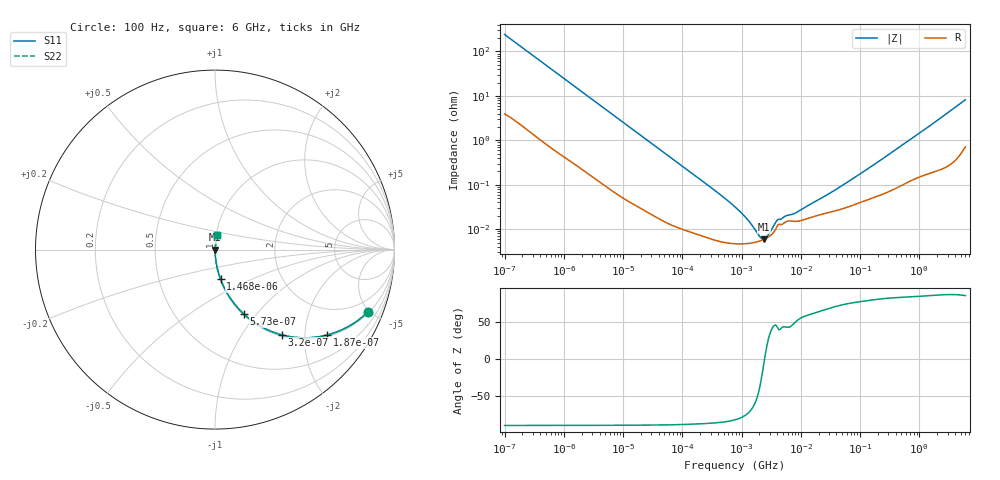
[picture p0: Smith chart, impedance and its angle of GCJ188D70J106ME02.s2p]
!Murata Part Number: GCJ188D70J106ME02
!These Parameters are Measured in Series Mode Connection
!Data Generated on Mar 13, 2026
!  o--ll--o
!Port1  Port2
!  o------o
!Operation Temp=25[degC], DC Bias Voltage=0[V]
!Freq. Start=100[Hz] Stop=6[GHz] 401[Steps]
# Hz S RI R 50
!Freq.(Hz) S11(Real) S11(Imag) S21(Real) S21(Imag) S12(Real) S12(Imag) S22(Real) S22(Imag)
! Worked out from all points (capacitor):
!   401 points, 100 Hz to 6 GHz, reference 50 ohm
!   read as one part in series: C = 6.56 uF near 109 Hz
!   lowest |Z| = 5.89 mohm at 2.373 MHz (marker M1)
!   series resonance near 2.443 MHz, so ESL is about 650 pH
!   S11 on the Smith chart (normalised r, x): 100 Hz: 1.08, -4.83; 187 Hz: 1.04, -2.60; 320 Hz: 1.03, -1.53; 573 Hz: 1.01, -0.86; 1.468 kHz: 1.01, -0.34; 6 GHz: 1.01, +0.16
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100  0.8497 -0.3494  0.1503 0.3494  0.1503 0.3494  0.8497 -0.3494
187  0.6266 -0.4752  0.3734 0.4752  0.3734 0.4752  0.6266 -0.4752
320  0.3713 -0.4748  0.6287 0.4748  0.6287 0.4748  0.3713 -0.4748
573  0.1601 -0.3585  0.8399 0.3585  0.8399 0.3585  0.1601 -0.3585
897  0.0745 -0.2542  0.9255 0.2542  0.9255 0.2542  0.0745 -0.2542
1468  0.0307 -0.1639  0.9693 0.1639  0.9693 0.1639  0.0307 -0.1639
2008  0.0174 -0.122  0.9826 0.122  0.9826 0.122  0.0174 -0.122
6433  0.00228 -0.0392  0.9977 0.0392  0.9977 0.0392  0.00228 -0.0392
40335  0.000212 -0.00641  0.9998 0.00641  0.9998 0.00641  0.000212 -0.00641
330837  5.84e-05 -0.000794  0.9999 0.000794  0.9999 0.000794  5.84e-05 -0.000794
774597  4.69e-05 -0.000313  1 0.000313  1 0.000313  4.69e-05 -0.000313
1108252  4.68e-05 -0.000194  1 0.000194  1 0.000194  4.68e-05 -0.000194
1658239  5.01e-05 -8.8e-05  0.9999 8.8e-05  0.9999 8.8e-05  5.01e-05 -8.8e-05
2372521  5.85e-05 -6.5e-06  0.9999 6.5e-06  0.9999 6.5e-06  5.85e-05 -6.5e-06
3103719  7.27e-05 5.46e-05  0.9999 -5.46e-05  0.9999 -5.46e-05  7.27e-05 5.46e-05
4246196  0.000129 0.000105  0.9999 -0.000105  0.9999 -0.000105  0.000129 0.000105
8311524  0.00015 0.000181  0.9999 -0.000181  0.9999 -0.000181  0.00015 0.000181
1.555665e7  0.000188 0.000335  0.9998 -0.000335  0.9998 -0.000335  0.000188 0.000335
4.764863e7  0.000281 0.000877  0.9997 -0.000877  0.9997 -0.000877  0.000281 0.000877
3.124326e8  0.00073 0.00485  0.9993 -0.00485  0.9993 -0.00485  0.00073 0.00485
1.873145e9  0.00265 0.026  0.9973 -0.026  0.9973 -0.026  0.00265 0.026
6e9  0.0135 0.0797  0.9865 -0.0797  0.9865 -0.0797  0.0135 0.0797
